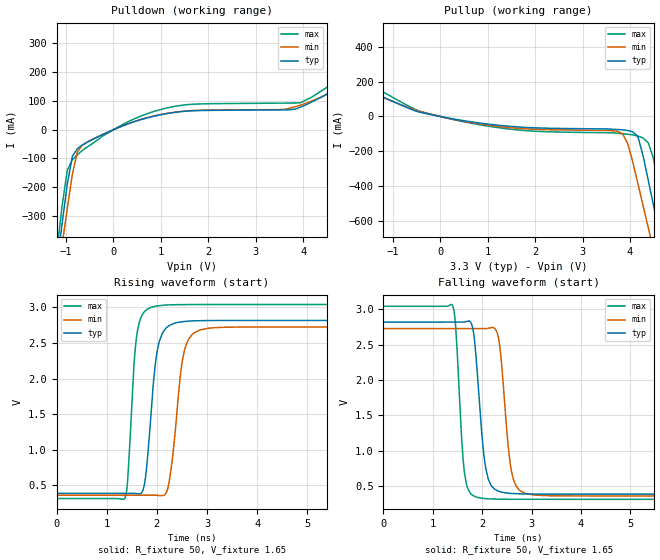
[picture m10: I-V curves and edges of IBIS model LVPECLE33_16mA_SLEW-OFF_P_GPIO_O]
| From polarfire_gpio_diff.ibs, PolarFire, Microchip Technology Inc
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|   Model LVPECLE33_16mA_SLEW-OFF_P_GPIO_O
[Model]   LVPECLE33_16mA_SLEW-OFF_P_GPIO_O
Model_type   Output
Polarity   Non-Inverting
Enable   Active-High
Vmeas =   1.65
Cref =   5p
Rref =   100
|   typ   min   max
C_comp_pullup   2.605e-12   2.605e-12   2.76e-12
C_comp_pulldown  2.605e-12   2.605e-12   2.76e-12
[Temperature Range]  25C   100C   -40C
[Voltage Range]  3.3   3.135   3.465
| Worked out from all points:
|   slope of the pulldown table from 0 to 0.495 V, typ, clamps not added: 16 ohm
|   slope of the pullup table from 0 to 0.495 V, typ, clamps not added: 20.7 ohm
|   rising waveform, R_fixture 50, V_fixture 1.65: 20-80 % time 181ps typ, 206ps min, 137ps max; typ from 0.389 V to 2.82 V
|   falling waveform, R_fixture 50, V_fixture 1.65: 20-80 % time 172ps typ, 174ps min, 130ps max; typ from 2.82 V to 0.389 V
[Pullup]
| Voltage   I(typ)   I(min)   I(max)
-3.3V     427mA      396.9mA    511.1mA
-433.1mV  24.19mA    29.02mA    29.79mA
1.444V    -55.61mA   -63.1mA    -71.57mA
3.733V    -74.42mA   -84.7mA    -95.53mA
3.95V     -79.97mA   -154.1mA   -101.6mA
4.058V    -87.8mA    -260.8mA   -104.9mA
4.166V    -114.9mA   -385.2mA   -111.7mA
4.383V    -363.8mA   -634.3mA   -149.9mA
4.491V    -503.8mA   -758.8mA   -237.6mA
4.708V    -784.1mA   -1.008A    -544.3mA
4.924V    -1.065A    -1.258A    -861.9mA
6.6V      -3.277A    -3.233A    -3.371A
[Pulldown]
| Voltage   I(typ)   I(min)   I(max)
-3.3V     -3.232A    -2.98A     -3.562A
-1.191V   -467.3mA   -525.2mA   -421mA
-1.083V   -327.3mA   -400.4mA   -264.9mA
-974.5mV  -190.3mA   -275.6mA   -141.6mA
-866.2mV  -92.32mA   -154.5mA   -104.5mA
-758mV    -65.3mA    -75.74mA   -86.44mA
-541.4mV  -42.49mA   -41.6mA    -58.54mA
1.238V    58.96mA    59.83mA    79.59mA
3.841V    72.16mA    80.37mA    93.04mA
4.708V    145.2mA    140.5mA    171.5mA
6.007V    310.5mA    287.8mA    365.3mA
6.6V      407.6mA    374.6mA    471.6mA
[Ramp]
dV/dt_r   1.45721/0.181254n  1.41779/0.205982n  1.63558/0.137202n
dV/dt_f   1.4572/0.171945n  1.41779/0.174191n  1.63558/0.129713n
R_load = 50
[Rising Waveform]
R_fixture = 50
V_fixture = 1.65
V_fixture_min = 1.5675
V_fixture_max = 1.7325
| Time   V(typ)   V(min)   V(max)
0s        389mV      363.2mV    315.5mV
1.362ns   388.9mV    363.4mV    320.2mV
1.59ns    385.3mV    363.5mV    2.557V
1.746ns   490.2mV    363.5mV    2.936V
1.867ns   1.347V     363.5mV    2.997V
2.101ns   2.625V     356.2mV    3.03V
2.261ns   2.752V     620.1mV    3.037V
2.554ns   2.804V     2.407V     3.04V
2.841ns   2.814V     2.679V     3.042V
10ns      2.818V     2.726V     3.041V
[Falling Waveform]
R_fixture = 50
V_fixture = 1.65
V_fixture_min = 1.5675
V_fixture_max = 1.7325
| Time   V(typ)   V(min)   V(max)
0s        2.818V     2.726V     3.041V
1.404ns   2.817V     2.726V     3.047V
1.464ns   2.817V     2.726V     2.749V
1.642ns   2.819V     2.725V     689.6mV
1.875ns   2.342V     2.725V     348.4mV
2.123ns   603.4mV    2.732V     322.8mV
2.346ns   426.9mV    2.533V     317.4mV
2.607ns   397.9mV    667.6mV    316.1mV
2.861ns   391.4mV    403.8mV    316mV
10ns      389mV      363.2mV    315.5mV
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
